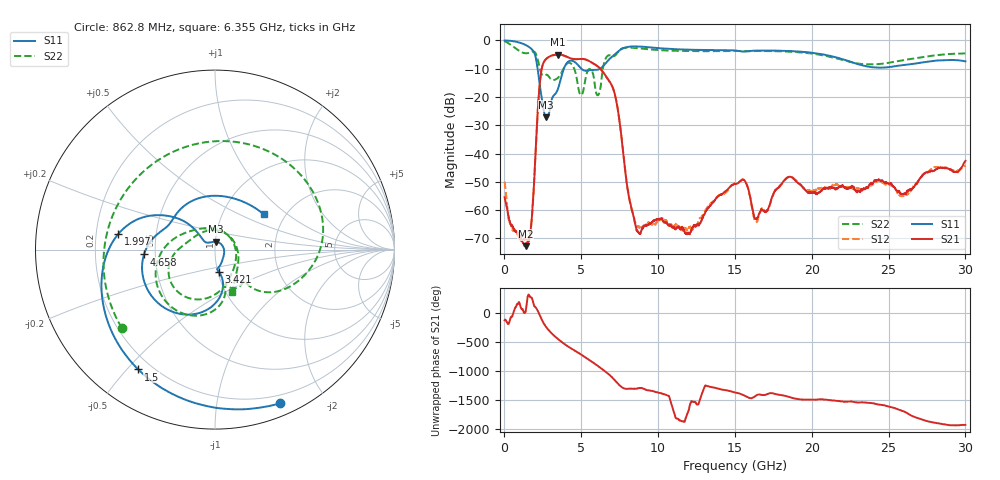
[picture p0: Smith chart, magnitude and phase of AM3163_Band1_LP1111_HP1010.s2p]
!Agilent Technologies,E8364B,MY43040894,A.07.50.67
!Agilent E8364B: A.07.50.67
!Date: Thursday, August 20, 2020 12:00:34
!Correction: S11(Full 2 Port(1,2))
!S21(Full 2 Port(1,2))
!S12(Full 2 Port(1,2))
!S22(Full 2 Port(1,2))
!S2P File: Measurements: S11, S21, S12, S22:
# Hz S  dB  R 50
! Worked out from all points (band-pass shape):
!   3201 points, 10 MHz to 30 GHz, reference 50 ohm
!   highest |S21| = -5.03 dB at 3.496 GHz (marker M1); lowest = -72.7 dB at 1.378 GHz (marker M2)
!   |S21| within 3 dB of the highest: 2.531 GHz to 5.739 GHz (3.208 GHz wide, 77.6 % of centre)
!   lowest |S11| = -27.2 dB at 2.709 GHz (marker M3), VSWR 1.09, Z = 50.1 + j4.37 ohm
!   |S11| at or under -10 dB: 2.157 GHz to 3.868 GHz (1.711 GHz wide, 56.8 % of centre); 5.003 GHz to 6.237 GHz (1.233 GHz wide, 21.9 % of centre)
!   |S22| runs from -19.4 to -0.3 dB; largest |S21 - S12| = 0.0029
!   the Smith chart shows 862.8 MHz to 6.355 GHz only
!   S11 on the Smith chart (normalised r, x): 862.8 MHz: 0.12, -1.50; 1.5 GHz: 0.15, -0.54; 1.997 GHz: 0.30, +0.07; 3.421 GHz: 1.01, -0.26; 4.658 GHz: 0.43, -0.03; 6.355 GHz: 1.56, +0.69
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1e7  -0.06 -5.1  -55.43 -123.3  -49.95 -157.7  -0.32 -12.0
8.628406e8  -0.64 -67.1  -67.89 152.9  -68.70 103.4  -3.37 -140.0
1.378294e9  -1.65 -111.0  -72.72 27.2  -70.23 20.1  -4.58 134.6
1.500128e9  -2.01 -122.6  -71.72 -83.0  -70.90 114.5  -4.54 112.8
1.996838e9  -5.26 170.8  -42.81 108.7  -42.70 108.2  -4.29 9.2
2.7091e9  -27.21 86.2  -6.61 121.2  -6.62 121.1  -12.20 -54.2
3.421362e9  -17.99 -80.1  -5.05 -74.5  -5.06 -74.5  -13.53 -74.3
3.496338e9  -16.95 -77.5  -5.03 -91.0  -5.05 -91.0  -13.20 -74.9
3.955559e9  -8.93 -102.3  -5.57 175.8  -5.58 176.0  -8.93 -96.2
4.65845e9  -8.03 -176.1  -6.68 58.7  -6.66 58.8  -12.20 167.7
5.014581e9  -10.06 160.4  -6.57 -0.4  -6.55 -0.5  -19.32 30.4
6.354759e9  -9.50 36.1  -10.76 112.5  -10.82 112.4  -11.82 -68.2
7.516872e9  -3.45 -102.4  -29.71 -174.5  -29.69 -173.4  -3.37 -170.3
8.613381e9  -2.16 172.9  -67.20 136.0  -65.56 133.5  -2.76 124.7
1.000979e10  -2.76 100.6  -63.29 66.5  -63.78 63.7  -3.45 65.7
1.227778e10  -3.36 9.7  -65.97 -91.9  -66.50 -114.8  -3.84 -14.9
1.5005e10  -3.58 -74.0  -50.71 67.8  -50.59 67.3  -3.79 -92.5
1.637329e10  -3.64 -104.6  -63.01 12.5  -64.16 173.6  -3.80 -125.9
2.000958e10  -4.39 162.7  -53.79 -54.4  -53.53 -53.9  -4.70 135.6
2.274617e10  -7.99 59.9  -51.90 -95.3  -52.43 -101.4  -7.94 20.4
2.500479e10  -9.50 -62.9  -50.63 -175.3  -50.77 -172.0  -7.96 -93.3
3e10  -7.42 104.8  -42.59 -133.5  -44.27 -134.7  -4.64 100.9
